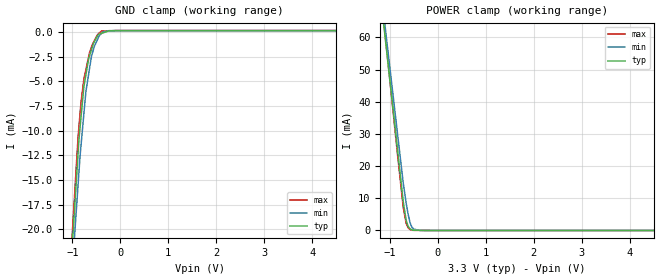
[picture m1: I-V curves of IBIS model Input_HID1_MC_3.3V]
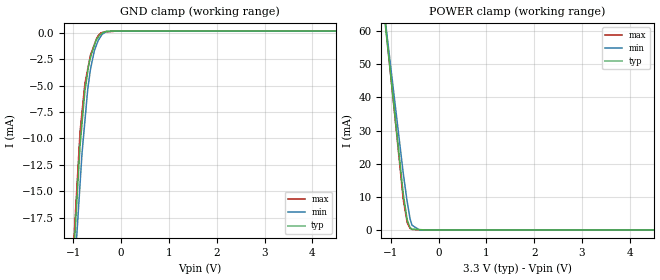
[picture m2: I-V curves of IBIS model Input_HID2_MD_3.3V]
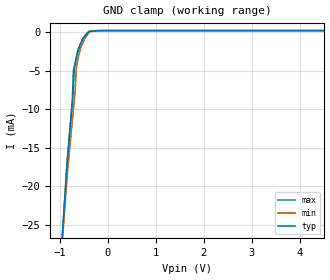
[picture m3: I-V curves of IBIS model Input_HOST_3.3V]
|Texas Instruments Incorporated
|Stereo Audio DAC w/ USB interface,
|Single-Ended Headphone Output and S/PDIF Output
| Marketing part#   Package-type   #pins/pkg drawing
|   PCM2704C   SSOP   28
[IBIS Ver]   4.0
[Comment Char] |_char
[File Name]   pcm2704c.ibs
[File Rev]   3.0
[Source]   Texas Instruments Incorporated.
   Analog-eLab, HPA
   12500 TI Blvd
   Dallas, TX -75243
[Date]   10-18-2004
[Notes]   Quality Check of this IBIS model: Model Passes IBIS Check
   Model parses into ICX IS. Simulation done with Hyperlynx.
   1. MIN TYP MAX information is based on Temprature and Voltage
   characteristics only.
[Disclaimer]
| This model is designed as an aid for customers of Texas Instruments.
| TI and its licensors and suppliers make no warranties, either expressed
| or implied, with respect to this  model, including the warranties of
| merchantability or fitness for a particular purpose.
| The model is provided solely on an "as is" basis. The entire risk as to
| its quality and performance is with the customer.
[Copyright]
| (C) Copyright 2011 Texas Instruments Incorporated. All rights reserved.
[Component] PCM2704C
[Manufacturer] TI
[Package]
| variable   typ   min   max
R_pkg  1.8006E-02  1.8006E-02  1.8006E-02
L_pkg  2.1607E-09  2.1607E-09  2.1607E-09
C_pkg  6.0021E-13  6.0021E-13  6.0021E-13
[Pin] signal_name  model_name  R_pin  L_pin C_pin
1   XTO   Output_XTO_3.3V   1.9723E-02  2.3076E-09  5.4618E-13
2   CK   Output_CK_3.3V   1.8868E-02  2.2076E-09  5.2250E-13
3   DT   BI_DT_3.3V   1.8028E-02  2.1092E-09  4.9923E-13
4   PSEL   Input_PSEL_3.3V   1.7205E-02  2.0129E-09  4.7644E-13
5   DOUT   Output_DOUT_3.3V   1.6401E-02  1.9189E-09  4.5419E-13
6   DGND   GND   1.5620E-02  1.8276E-09  4.3257E-13
7   VDD   POWER   1.4866E-02  1.7393E-09  4.1168E-13
8   D-   USB_3.3V   1.4866E-02  1.7393E-09  4.1168E-13
9   D+   USB_3.3V   1.5620E-02  1.8276E-09  4.3257E-13
10  VBUS   POWER   1.6401E-02  1.9189E-09  4.5419E-13
11  ZGND   GND   1.7205E-02  2.0129E-09  4.7644E-13
12  AGNDL   GND   1.8028E-02  2.1092E-09  4.9923E-13
13  VCCL   POWER   1.8868E-02  2.2076E-09  5.2250E-13
14  VoutL   NC   1.9723E-02  2.3076E-09  5.4618E-13
15  VoutR   NC   1.9723E-02  2.3076E-09  5.4618E-13
16  VCCR   POWER   1.8868E-02  2.2076E-09  5.2250E-13
17  AGNDR   GND   1.8028E-02  2.1092E-09  4.9923E-13
18  VCOM   POWER   1.7205E-02  2.0129E-09  4.7644E-13
19  PGND   GND   1.6401E-02  1.9189E-09  4.5419E-13
20  VCCP   POWER   1.5620E-02  1.8276E-09  4.3257E-13
21  HOST   Input_HOST_3.3V   1.4866E-02  1.7393E-09  4.1168E-13
22  HID0   Input_HID0_MS_3.3V  1.4866E-02  1.7393E-09  4.1168E-13
23  HID1   Input_HID1_MC_3.3V  1.5620E-02  1.8276E-09  4.3257E-13
24  HID2   Input_HID2_MD_3.3V  1.6401E-02  1.9189E-09  4.5419E-13
25  TEST1   Input_TEST1_3.3V   1.7205E-02  2.0129E-09  4.7644E-13
26  TEST0   Input_TEST0_3.3V   1.8028E-02  2.1092E-09  4.9923E-13
27  _SSPND   Output_SSPND_3.3V   1.8868E-02  2.2076E-09  5.2250E-13
28  XTI   Input_XTI_3.3V   1.9723E-02  2.3076E-09  5.4618E-13
| Models and submodels in the file (14): Input_HID1_MC_3.3V (Input), Input_HID2_MD_3.3V (Input), Input_HID0_MS_3.3V (Input), Input_HOST_3.3V (Input), Input_PSEL_3.3V (Input), Input_TEST0_3.3V (Input), Input_TEST1_3.3V (Input), Input_XTI_3.3V (Input), Output_CK_3.3V (Output), Output_DOUT_3.3V (Output), BI_DT_3.3V (I/O), Output_SSPND_3.3V (Output), Output_XTO_3.3V (Output), USB_3.3V (I/O)
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[Model] Input_HID1_MC_3.3V
Model_type Input
Vinl  = 800.000mV
Vinh  = 2.00000V
C_comp  2.00000pF 2.00000pF 2.00000pF
| variable   typ   min   max
[Voltage Range]   3.30000V  3.00000V  3.60000V
[POWER Clamp Reference]  3.30000V  3.00000V  3.60000V
[GND Clamp Reference]   0.00000V  0.00000V  0.00000V
[Temperature Range]   25   85   -25
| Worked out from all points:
|   GND clamp passes 1 mA (typ) near -0.55 V on its own axis
|   POWER clamp passes 1 mA (typ) near -0.60 V on its own axis
[GND Clamp]
-3.3V     -198.8mA   -187mA     -207.8mA
-881.1mV  -12.31mA   -15.49mA   -10.64mA
-861.1mV  -10.77mA   -14.08mA   -9.489mA
-820.8mV  -8.675mA   -11.56mA   -7.169mA
-760.1mV  -5.523mA   -8.271mA   -4.759mA
-719.6mV  -4.376mA   -6.078mA   -3.836mA
-659mV    -2.662mA   -4.201mA   -2.457mA
-603.2mV  -1.796mA   -2.471mA   -1.534mA
-461.8mV  -223.6uA   -588.8uA   -189.1uA
-390.9mV  -110.6uA   -114.1uA   123uA
-110.6mV  144.4uA    171uA      162.2uA
6.6V      144.4uA    171uA      168.5uA
[POWER Clamp]
-3.3V     358.2mA    346.1mA    380.2mA
-1.039V   52.01mA    55.59mA    52.39mA
-842.3mV  25.32mA    30.27mA    23.83mA
-721.1mV  8.907mA    14.7mA     7.145mA
-660.2mV  3.154mA    8.48mA     2.208mA
-619.9mV  1.299mA    5.074mA    839uA
-579.2mV  517uA      2.386mA    287uA
-538.6mV  143.5uA    950.4uA    53uA
-498mV    121.8uA    421.7uA    47.85uA
-381.7mV  59.89uA    0A         33.08uA
6.6V      0A         0A         0A
[Model] Input_HID2_MD_3.3V
Model_type Input
Vinl  = 800.000mV
Vinh  = 2.00000V
C_comp  2.00000pF 2.00000pF 2.00000pF
| variable   typ   min   max
[Voltage Range]   3.30000V  3.00000V  3.60000V
[POWER Clamp Reference]  3.30000V  3.00000V  3.60000V
[GND Clamp Reference]   0.00000V  0.00000V  0.00000V
[Temperature Range]   25   85   -25
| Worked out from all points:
|   GND clamp passes 1 mA (typ) near -0.55 V on its own axis
|   POWER clamp passes 1 mA (typ) near -0.61 V on its own axis
[GND Clamp]
-3.3V     -202.3mA   -188.4mA   -204.3mA
-861.2mV  -10.72mA   -14.36mA   -9.41mA
-820.9mV  -8.663mA   -11.49mA   -7.586mA
-760.1mV  -5.554mA   -8.402mA   -4.835mA
-699.5mV  -3.669mA   -5.325mA   -3.426mA
-643.8mV  -2.39mA    -3.477mA   -2.13mA
-562.3mV  -1.186mA   -1.697mA   -1.114mA
-502mV    -524.1uA   -970uA     -443.3uA
-421mV    -152uA     -289.9uA   1.582uA
-310.9mV  131.6uA    135.8uA    112.4uA
-181.8mV  165.3uA    158.2uA    136.9uA
6.6V      176.1uA    158.9uA    160.8uA
[POWER Clamp]
-3.3V     358.5mA    330.7mA    375.2mA
-1.039V   51.39mA    53.61mA    51.84mA
-741.1mV  10.88mA    17.07mA    9.188mA
-660.1mV  3.071mA    8.621mA    2.296mA
-599.6mV  727.7uA    3.402mA    494.6uA
-559.1mV  265uA      1.442mA    152.2uA
-402.1mV  116.2uA    5.961uA    32.75uA
6.6V      0A         0A         0A
[Model] Input_HOST_3.3V
Model_type Input
Vinl  = 800.000mV
Vinh  = 2.00000V
C_comp  2.00000pF 2.00000pF 2.00000pF
| variable   typ   min   max
[Voltage Range]   3.30000V  3.00000V  3.60000V
[POWER Clamp Reference]  3.30000V  3.00000V  3.60000V
[GND Clamp Reference]   0.00000V  0.00000V  0.00000V
[Temperature Range]   25   85   -25
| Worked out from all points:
|   GND clamp passes 1 mA (typ) near -0.53 V on its own axis
[GND Clamp]
-3.3V     -243.7mA   -224.9mA   -258.1mA
-861.2mV  -18.2mA    -19.8mA    -17.84mA
-840.9mV  -16.33mA   -18.09mA   -16.3mA
-739.7mV  -9.137mA   -11.46mA   -8.638mA
-719.7mV  -7.713mA   -10.15mA   -5.058mA
-699.5mV  -4.792mA   -8.821mA   -4.473mA
-679.1mV  -4.138mA   -7.485mA   -3.884mA
-659mV    -3.493mA   -4.781mA   -3.302mA
-623.6mV  -2.607mA   -3.468mA   -2.28mA
-562.2mV  -1.505mA   -1.988mA   -1.389mA
-380.8mV  64.81uA    5.095uA    131.8uA
6.6V      188.4uA    189.4uA    203.1uA
[POWER Clamp]
| Voltage   I(typ)   I(min)   I(max)
-3.6V     0A         0A         0A
-3.5V     0A         0A         0A
-3.4V     0A         0A         0A
7.2V      0A         0A         0A
